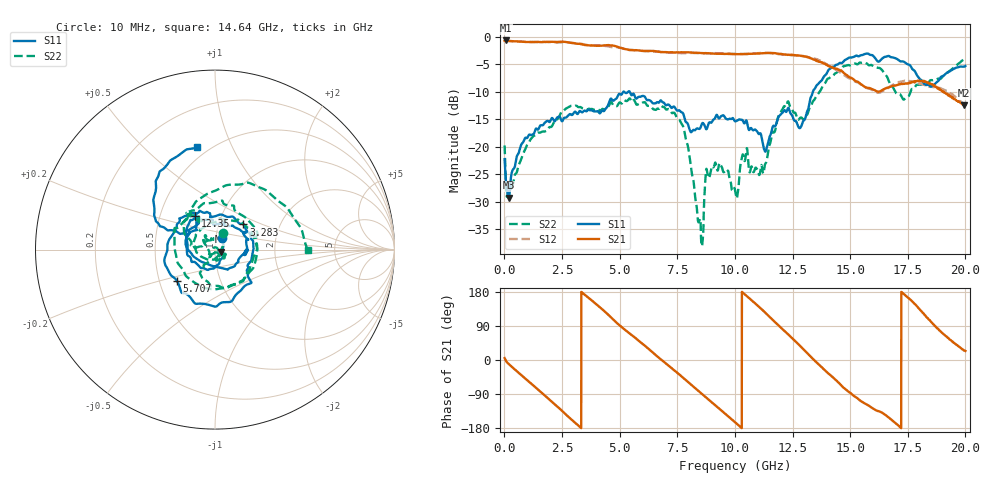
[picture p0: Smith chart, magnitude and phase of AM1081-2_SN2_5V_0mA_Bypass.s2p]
!Agilent Technologies,E8364B,MY43040894,A.07.50.67
!Agilent E8364B: A.07.50.67
!Date: Wednesday, June 23, 2021 07:36:05
!Correction: S11(Full 2 Port(1,2))
!S21(Full 2 Port(1,2))
!S12(Full 2 Port(1,2))
!S22(Full 2 Port(1,2))
!S2P File: Measurements: S11, S21, S12, S22:
# Hz S  dB  R 50
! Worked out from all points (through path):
!   3201 points, 10 MHz to 20 GHz, reference 50 ohm
!   highest |S21| = -0.66 dB at 72.47 MHz (marker M1); lowest = -12.5 dB at 19.95 GHz (marker M2)
!   group delay of S21, straight-line fit = 147 ps
!   lowest |S11| = -29.3 dB at 184.9 MHz (marker M3), VSWR 1.07, Z = 53.3 - j1.24 ohm
!   |S11| at or under -10 dB: start of sweep to 5.157 GHz; 5.196 GHz to 5.37 GHz (173.7 MHz wide, 3.29 % of centre); 5.44 GHz to 13.38 GHz (7.944 GHz wide, 84.4 % of centre)
!   |S22| runs from -38.1 to -4.0 dB; largest |S21 - S12| = 0.031
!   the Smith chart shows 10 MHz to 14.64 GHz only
!   S11 on the Smith chart (normalised r, x): 10 MHz: 1.08, +0.14; 3.283 GHz: 1.31, +0.39; 5.707 GHz: 0.62, -0.24; 12.35 GHz: 0.75, +0.30; 14.64 GHz: 0.44, +0.74
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1e7  -22.26 57.3  -0.73 5.0  -0.69 4.4  -19.76 65.3
7.246875e7  -26.64 15.5  -0.66 -2.8  -0.68 -2.8  -27.52 17.1
1.849125e8  -29.27 -19.7  -0.75 -10.4  -0.77 -10.3  -27.07 -30.1
1.752878e9  -15.62 170.8  -0.92 -93.6  -0.92 -94.0  -17.22 117.5
3.283362e9  -13.50 41.5  -1.29 -177.2  -1.26 -176.8  -12.77 -46.2
3.345831e9  -13.70 35.0  -1.31 179.3  -1.29 180.0  -12.88 -51.6
4.638934e9  -11.26 -43.3  -1.59 111.7  -1.87 111.8  -11.87 151.8
5.70715e9  -11.22 -140.2  -2.42 56.9  -2.42 56.8  -12.19 63.4
6.675416e9  -11.96 143.6  -2.69 7.1  -2.71 7.8  -13.07 -33.4
7.737384e9  -13.84 97.8  -2.80 -46.0  -2.98 -45.6  -16.14 -122.8
8.530738e9  -16.27 71.6  -2.95 -87.5  -2.99 -86.5  -36.62 28.5
9.074216e9  -15.03 39.3  -3.05 -115.7  -2.98 -114.9  -23.72 -24.4
1.0005e10  -15.37 -2.6  -3.13 -164.1  -3.08 -164.0  -27.88 -143.2
1.235382e10  -13.21 120.3  -3.27 65.1  -3.33 65.8  -12.20 127.6
1.334083e10  -10.59 157.2  -3.97 5.7  -3.87 6.4  -12.21 123.8
1.464018e10  -4.77 99.9  -6.27 -68.9  -6.72 -69.0  -5.71 -0.2
1.563968e10  -3.12 25.7  -9.11 -114.9  -9.15 -114.7  -4.71 -62.2
1.667042e10  -3.47 -14.3  -9.20 -151.6  -9.20 -148.5  -8.03 -137.5
1.758246e10  -5.11 -51.1  -8.37 160.5  -8.06 157.3  -10.45 75.1
1.851949e10  -9.04 -150.8  -8.63 100.2  -9.11 103.4  -7.88 -14.3
1.995002e10  -5.42 100.0  -12.48 25.0  -12.30 22.3  -4.08 -164.8
2e10  -5.31 97.2  -12.39 23.8  -12.31 20.6  -4.08 -167.3
